(* Logix 5000 AddOnInstructionDefinition export GracoCore_DecodeDateTime; software revision 32.04 *)

TYPE GracoCore_TypeDateTime :
STRUCT
   year : DINT;   // year (yyyy)
   month : DINT;   // month (1=January, 2=February...12=December)
   dayOfMonth : DINT;   // day of the month (1-31)
   dayOfWeek : DINT;   // day of the week (1=Monday, 2=Tuesday...7=Sunday)
   hour : DINT;   // hour (0-23)
   min : DINT;   // min (0-59)
   sec : DINT;   // second (0-59)
END_STRUCT
END_TYPE

TYPE GracoPd2kDual_TypePd2kDualStatus :
STRUCT
   gunTriggerStatus1 : BOOL;   // gun 1 trigger status (1 = on)
   gunTriggerStatus2 : BOOL;   // gun 2 trigger status (1 = on)
   mixUnit1 : GracoPd2kDual_TypePd2kMixUnitStatus;   // mix unit 1
   mixUnit2 : GracoPd2kDual_TypePd2kMixUnitStatus;   // mix unit 2
   pump1 : GracoPd2kDual_TypePd2kPump;   // pump 1
   pump2 : GracoPd2kDual_TypePd2kPump;   // pump 2
   pump3 : GracoPd2kDual_TypePd2kPump;   // pump 3
   pump4 : GracoPd2kDual_TypePd2kPump;   // pump 4
   dcsReturn0 : DINT;   // DCS return 0
   dcsReturn1 : DINT;   // DCS return 1
   dcsReturn2 : DINT;   // DCS return 2
   dcsReturn3 : DINT;   // DCS return 3
   dcsReturn4 : DINT;   // DCS return 4
   dcsReturn5 : DINT;   // DCS return 5
   dcsReturn6 : DINT;   // DCS return 6
   dcsReturn7 : DINT;   // DCS return 7
   dcsReturn8 : DINT;   // DCS return 8
   dcsAck : DINT;   // DCS acknowledge
END_STRUCT
END_TYPE

TYPE GracoPd2kDual_TypePd2kMixUnitStatus :
STRUCT
   eventFlag : BOOL;   // event flag
   standby : BOOL;   // in standby
   interlockStatus : BOOL;   // interlock status
   systemMode : DINT;   // system mode
   systemModeFlags : GracoPd2kDual_TypePd2kSystemModeFlags;   // system mode flags
   actualMixFlow : DINT;   // actual mix flow (cc/min)
   actualMixRatio : DINT;   // actual mix ratio
   actualPotLifeRemaining : DINT;   // actual pot life remaining
   activeRecipeNum : DINT;   // active recipe number
   activeMaterialA : DINT;   // active material A
   activeMaterialB : DINT;   // active material B
   activeFlushSeqA : DINT;   // active flush sequence A
   activeFlushSeqB : DINT;   // active flush sequence B
   activeRatioSP : DINT;   // active ratio SP
   activePotLifeSP : DINT;   // active pot life SP
   activeJobNum : DINT;   // active job number
   jobSprayVolA : DINT;   // job sprayed volume A (cc)
   jobSprayVolB : DINT;   // job sprayed volume B (cc)
   jobSolventVol : DINT;   // job solvent volume used (cc)
END_STRUCT
END_TYPE

TYPE GracoPd2kDual_TypePd2kPump :
STRUCT
   status : DINT;   // pump status
   statusFlags : GracoPd2kDual_TypePd2kPumpStatusFlags;   // pump status flags
   actualMaterial : DINT;   // actual material number
   actualFlowRate : DINT;   // actual flow rate (cc/min)
   actualFluidPres : DINT;   // actual fluid pressure (psi)
END_STRUCT
END_TYPE

TYPE GracoPd2kDual_TypePd2kPumpStatusFlags :
STRUCT
   off : BOOL;   // off
   standby : BOOL;   // in standby
   busy : BOOL;   // busy
   flushing : BOOL;   // flushing
   priming : BOOL;   // priming
END_STRUCT
END_TYPE

TYPE GracoPd2kDual_TypePd2kSystemModeFlags :
STRUCT
   pumpOff : BOOL;   // pump off
   colorChange : BOOL;   // color change enabled
   colorChangePurgeA : BOOL;   // color change purging component A
   colorChangePurgeB : BOOL;   // color change purging component B
   colorChangeFilling : BOOL;   // color change filling
   mixFill : BOOL;   // mix fill
   mix : BOOL;   // mixing
   mixIdle : BOOL;   // mix idle
   purgeA : BOOL;   // purging component A
   purgeB : BOOL;   // purging component B
   standbyMixReady : BOOL;   // standby mix ready
   standbyFillReady : BOOL;   // standby fill ready
   standbyMixNotReady : BOOL;   // standby mix not ready
   standbyAlarm : BOOL;   // standby alarm
   lineFillingFlushing : BOOL;   // line is filling or flushing
   pumpPrimeFlush : BOOL;   // pump is priming or flushing
   maintCalibration : BOOL;   // maintenance/calibration
   mixSolventPush : BOOL;   // mix solvent push
END_STRUCT
END_TYPE

TYPE STRING4 :   // string type
STRUCT
   LEN : DINT;
   DATA : SINT[4];
END_STRUCT
END_TYPE

TYPE STRING9 :   // string type
STRUCT
   LEN : DINT;
   DATA : SINT[9];
END_STRUCT
END_TYPE

ADD_ON_INSTRUCTION GracoCore_DecodeDateTime   (* revision 1.0 *)
// Help:
// Convert from Graco-formatted date and time data into a UDT.
VAR_IN_OUT
   dateSource : DINT; {required}
   timeSource : DINT; {required}
   dateTimeDest : GracoCore_TypeDateTime; {required}
END_VAR
VAR
   buffer : DINT; {access None}
END_VAR

ROUTINE Logic   (* ladder *)
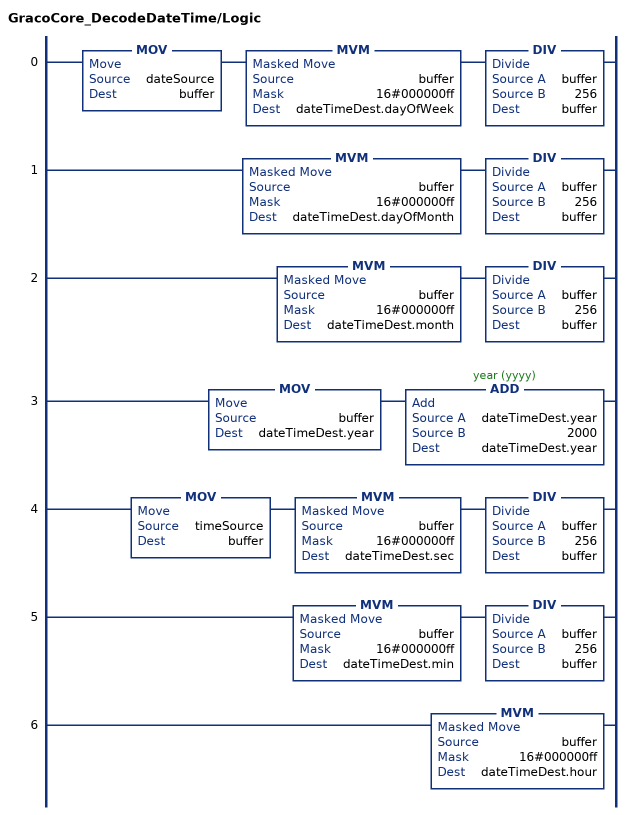
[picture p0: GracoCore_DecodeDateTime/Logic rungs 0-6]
   0: MOV(dateSource,buffer)MVM(buffer,16#000000ff,dateTimeDest.dayOfWeek)DIV(buffer,256,buffer);
   1: MVM(buffer,16#000000ff,dateTimeDest.dayOfMonth)DIV(buffer,256,buffer);
   2: MVM(buffer,16#000000ff,dateTimeDest.month)DIV(buffer,256,buffer);
   3: MOV(buffer,dateTimeDest.year)ADD(dateTimeDest.year,2000,dateTimeDest.year);
   4: MOV(timeSource,buffer)MVM(buffer,16#000000ff,dateTimeDest.sec)DIV(buffer,256,buffer);
   5: MVM(buffer,16#000000ff,dateTimeDest.min)DIV(buffer,256,buffer);
   6: MVM(buffer,16#000000ff,dateTimeDest.hour);
END_ROUTINE
END_ADD_ON_INSTRUCTION

ADD_ON_INSTRUCTION GracoCore_DecodeEventCode   (* revision 1.0 *)
// Help:
// Parses an event code String (max 4 characters) into a series of ASCII values stored in DINTs. These can then be written to a Graco CGM.
VAR_IN_OUT
   source : DINT; {required}
   dest : STRING4; {required}
END_VAR
VAR
   buffer : DINT; {access None}
END_VAR

ROUTINE Logic   (* ladder *)
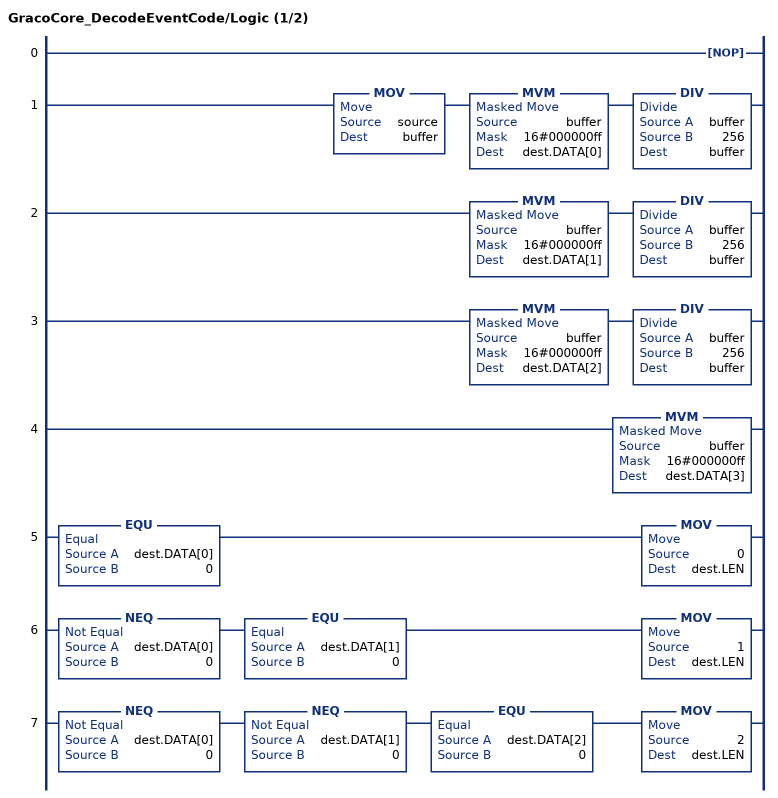
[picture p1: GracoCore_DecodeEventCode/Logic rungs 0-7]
   0: NOP();
   1: MOV(source,buffer)MVM(buffer,16#000000ff,dest.DATA[0])DIV(buffer,256,buffer);
   2: MVM(buffer,16#000000ff,dest.DATA[1])DIV(buffer,256,buffer);
   3: MVM(buffer,16#000000ff,dest.DATA[2])DIV(buffer,256,buffer);
   4: MVM(buffer,16#000000ff,dest.DATA[3]);
   5: EQU(dest.DATA[0],0)MOV(0,dest.LEN);
   6: NEQ(dest.DATA[0],0)EQU(dest.DATA[1],0)MOV(1,dest.LEN);
   7: NEQ(dest.DATA[0],0)NEQ(dest.DATA[1],0)EQU(dest.DATA[2],0)MOV(2,dest.LEN);
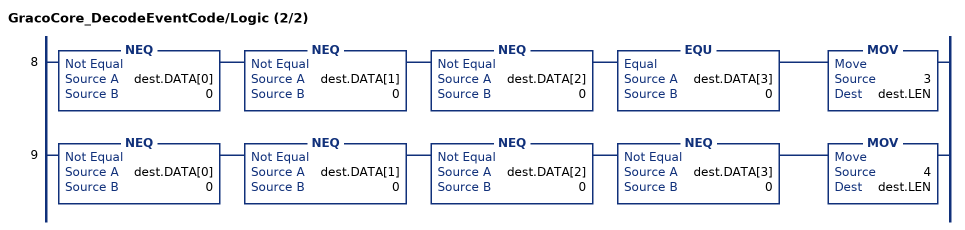
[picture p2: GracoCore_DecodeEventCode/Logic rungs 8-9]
   8: NEQ(dest.DATA[0],0)NEQ(dest.DATA[1],0)NEQ(dest.DATA[2],0)EQU(dest.DATA[3],0)MOV(3,dest.LEN);
   9: NEQ(dest.DATA[0],0)NEQ(dest.DATA[1],0)NEQ(dest.DATA[2],0)NEQ(dest.DATA[3],0)MOV(4,dest.LEN);
END_ROUTINE
END_ADD_ON_INSTRUCTION

ADD_ON_INSTRUCTION GracoPd2kDual_SendDCS   (* revision 1.0 *)
// Help:
// Sends a dynamic command structure (DCS) to the PD2K system.
// For more information about DCS commands, see the system operation manual.
// State Codes:
// * 0000 (IDLE) - Idle
// * 1000 (BUSY) - Busy
// * 2000 (DONE) - Done
// * 4000 (ABORT) - Command overwritten by another process
// * 8000 (ERROR) - Invalid command ID
// * 8001 (ERROR) - Timeout waiting for DCS registers
// * 8002 (ERROR) - Command unsuccessful
VAR_IN_OUT
   io_moduleStatus : DINT[62]; {required}   // Data from device to PLC
   io_moduleCmds : DINT[30]; {required}   // Data from PLC to device
END_VAR
VAR_INPUT
   i_execute : BOOL; {visible}   // Execute command
   i_cmdID : DINT; {visible}   // Command ID number
   i_arg0 : DINT; {visible}   // Argument 0
   i_arg1 : DINT; {visible}   // Argument 1
   i_arg2 : DINT; {visible}   // Argument 2
   i_arg3 : DINT; {visible}   // Argument 3
   i_arg4 : DINT; {visible}   // Argument 4
   i_arg5 : DINT; {visible}   // Argument 5
   i_arg6 : DINT; {visible}   // Argument 6
   i_arg7 : DINT; {visible}   // Argument 7
   i_arg8 : DINT; {visible}   // Argument 8
END_VAR
VAR_OUTPUT
   o_return0 : DINT; {access Read Only, visible}   // Return 0
   o_return1 : DINT; {access Read Only, visible}   // Return 1
   o_return2 : DINT; {access Read Only, visible}   // Return 2
   o_return3 : DINT; {access Read Only, visible}   // Return 3
   o_return4 : DINT; {access Read Only, visible}   // Return 4
   o_return5 : DINT; {access Read Only, visible}   // Return 5
   o_return6 : DINT; {access Read Only, visible}   // Return 6
   o_return7 : DINT; {access Read Only, visible}   // Return 7
   o_return8 : DINT; {access Read Only, visible}   // Return 8
   o_done : BOOL; {access Read Only, visible}   // Done flag
   o_busy : BOOL; {access Read Only, visible}   // Busy flag
   o_aborted : BOOL; {access Read Only, visible}   // Aborted flag
   o_error : BOOL; {access Read Only, visible}   // Error flag
   o_state : DINT; {access Read Only, visible}   // Command state
END_VAR
VAR
   _resetArgsTmr : TIMER := (PRE := 100); {access None}   // Reset arguments delay timer
   _inUseTmr : TIMER := (PRE := 5000); {access None}   // Register in use timer
   _sendArgsTmr : TIMER := (PRE := 100); {access None}   // Send arguments timer
   rateLimitTmr : TIMER := (PRE := 250); {access None}   // Rate limit timer
   cmdTimeoutTmr : TIMER := (PRE := 5000); {access None}   // Command timeout timer
   state_checkDcsReg : DINT; {access None}
   state_clearArgs : DINT; {access None}
   state_setArgs : DINT; {access None}
   state_setCmdID : DINT; {access None}
   state_awaitAck : DINT; {access None}
   state_rateLimit : DINT; {access None}
   state_done : DINT; {access None}
   state_aborted : DINT; {access None}
   state_invalidCmdID : DINT; {access None}
   state_dcsRegInUse : DINT; {access None}
   state_ackError : DINT; {access None}
   state_ackTimeout : DINT; {access None}
   initConfigValsDone : BOOL; {access None}
   _nextState : DINT; {access None}
   dcsRegAvailable : BOOL; {access None}
   _cmdID : DINT; {access None}
   execute_ons : BOOL; {access None}
END_VAR

ROUTINE Logic   (* ladder *)
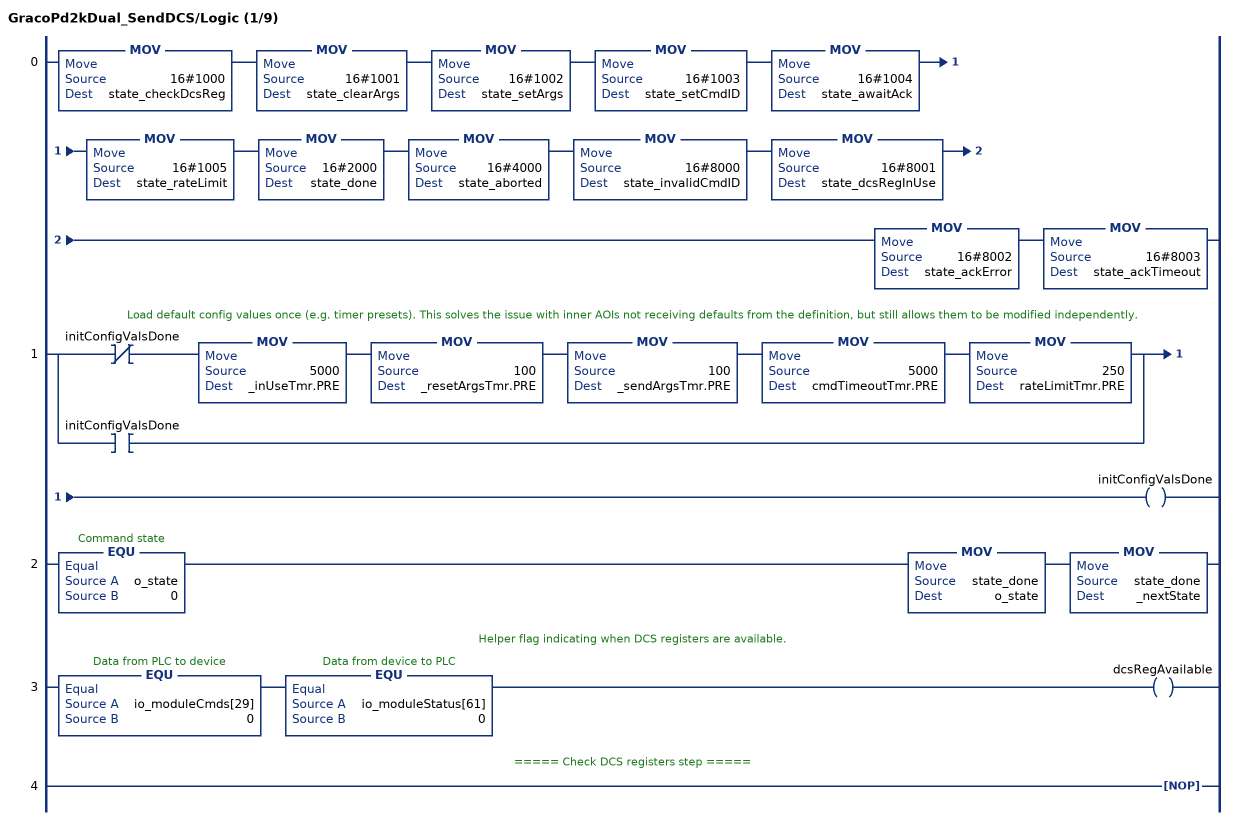
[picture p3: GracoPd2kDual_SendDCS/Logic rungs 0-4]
   0: MOV(16#1000,state_checkDcsReg)MOV(16#1001,state_clearArgs)MOV(16#1002,state_setArgs)MOV(16#1003,state_setCmdID)MOV(16#1004,state_awaitAck)MOV(16#1005,state_rateLimit)MOV(16#2000,state_done)MOV(16#4000,state_aborted)MOV(16#8000,state_invalidCmdID)MOV(16#8001,state_dcsRegInUse)MOV(16#8002,state_ackError)MOV(16#8003,state_ackTimeout);
   // Load default config values once (e.g. timer presets). This solves the issue with inner AOIs not receiving defaults from the definition, but still allows them to be modified independently.
   1: [XIO(initConfigValsDone) MOV(5000,_inUseTmr.PRE) MOV(100,_resetArgsTmr.PRE) MOV(100,_sendArgsTmr.PRE) MOV(5000,cmdTimeoutTmr.PRE) MOV(250,rateLimitTmr.PRE) ,XIC(initConfigValsDone) ]OTE(initConfigValsDone);
   2: EQU(o_state,0)MOV(state_done,o_state)MOV(state_done,_nextState);
   // Helper flag indicating when DCS registers are available.
   3: EQU(io_moduleCmds[29],0)EQU(io_moduleStatus[61],0)OTE(dcsRegAvailable);
   // ===== Check DCS registers step =====
   4: NOP();
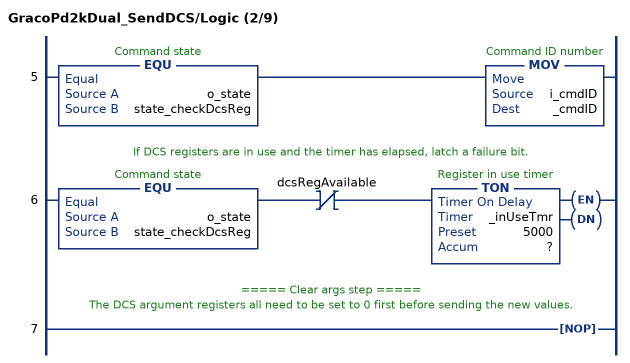
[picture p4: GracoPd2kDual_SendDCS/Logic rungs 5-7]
   5: EQU(o_state,state_checkDcsReg)MOV(i_cmdID,_cmdID);
   // If DCS registers are in use and the timer has elapsed, latch a failure bit.
   6: EQU(o_state,state_checkDcsReg)XIO(dcsRegAvailable)TON(_inUseTmr,?,?);
   // ===== Clear args step =====
   // The DCS argument registers all need to be set to 0 first before sending the new values.
   7: NOP();
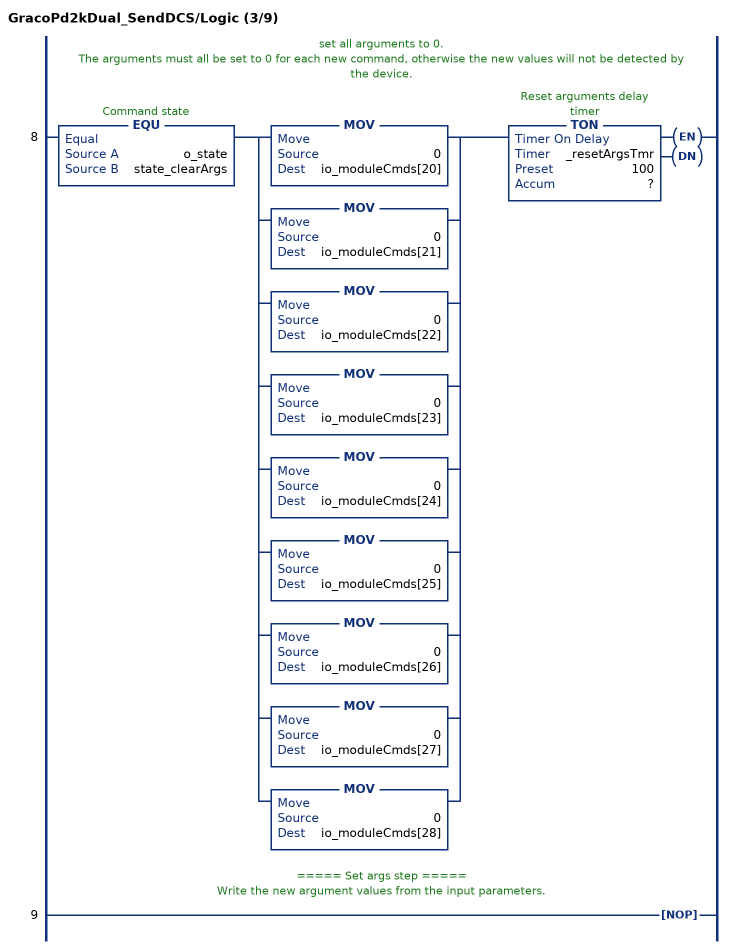
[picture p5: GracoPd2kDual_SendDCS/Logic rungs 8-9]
   // set all arguments to 0.
   // 		The arguments must all be set to 0 for each new command, otherwise the new values will not be detected by the device.
   8: EQU(o_state,state_clearArgs)[MOV(0,io_moduleCmds[20]) ,MOV(0,io_moduleCmds[21]) ,MOV(0,io_moduleCmds[22]) ,MOV(0,io_moduleCmds[23]) ,MOV(0,io_moduleCmds[24]) ,MOV(0,io_moduleCmds[25]) ,MOV(0,io_moduleCmds[26]) ,MOV(0,io_moduleCmds[27]) ,MOV(0,io_moduleCmds[28]) ]TON(_resetArgsTmr,?,?);
   // ===== Set args step =====
   // Write the new argument values from the input parameters.
   9: NOP();
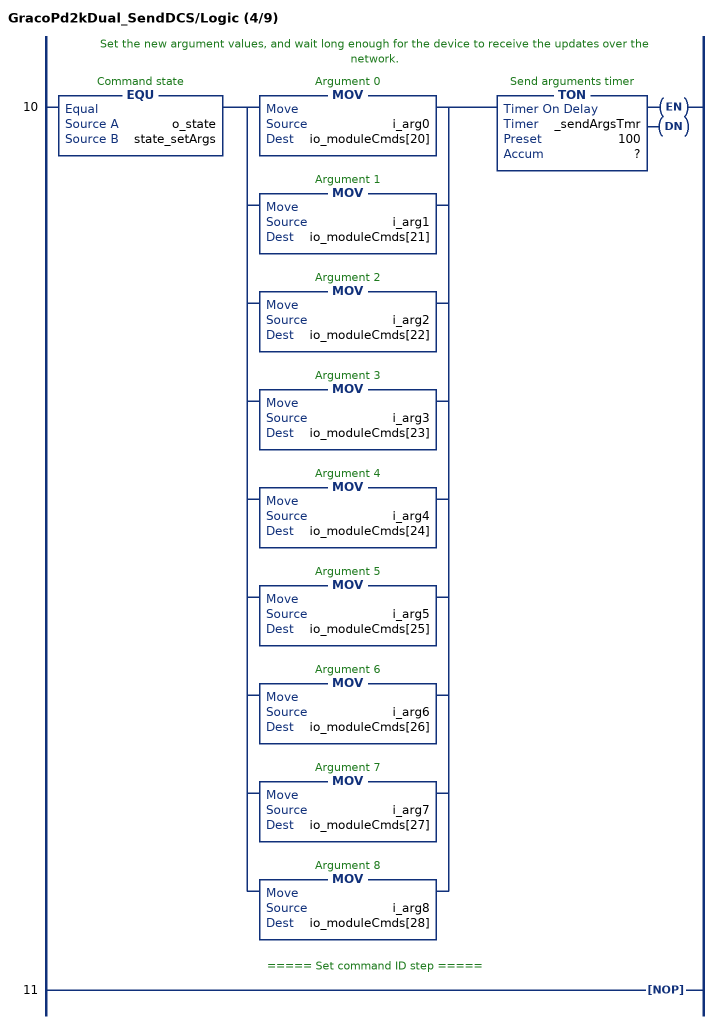
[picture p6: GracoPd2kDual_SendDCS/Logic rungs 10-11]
   // Set the new argument values, and wait long enough for the device to receive the updates over the network.
   10: EQU(o_state,state_setArgs)[MOV(i_arg0,io_moduleCmds[20]) ,MOV(i_arg1,io_moduleCmds[21]) ,MOV(i_arg2,io_moduleCmds[22]) ,MOV(i_arg3,io_moduleCmds[23]) ,MOV(i_arg4,io_moduleCmds[24]) ,MOV(i_arg5,io_moduleCmds[25]) ,MOV(i_arg6,io_moduleCmds[26]) ,MOV(i_arg7,io_moduleCmds[27]) ,MOV(i_arg8,io_moduleCmds[28]) ]TON(_sendArgsTmr,?,?);
   // ===== Set command ID step =====
   11: NOP();
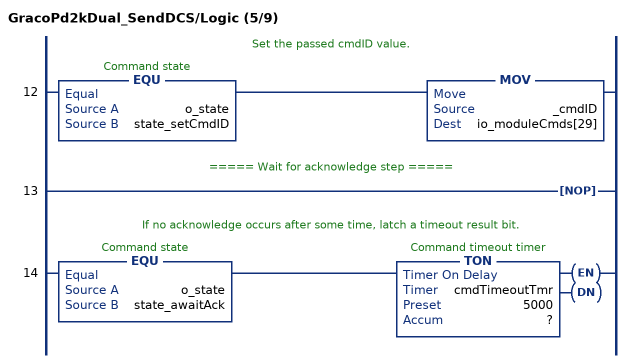
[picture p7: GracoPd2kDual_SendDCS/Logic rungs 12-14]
   // Set the passed cmdID value.
   12: EQU(o_state,state_setCmdID)MOV(_cmdID,io_moduleCmds[29]);
   // ===== Wait for acknowledge step =====
   13: NOP();
   // If no acknowledge occurs after some time, latch a timeout result bit.
   14: EQU(o_state,state_awaitAck)TON(cmdTimeoutTmr,?,?);
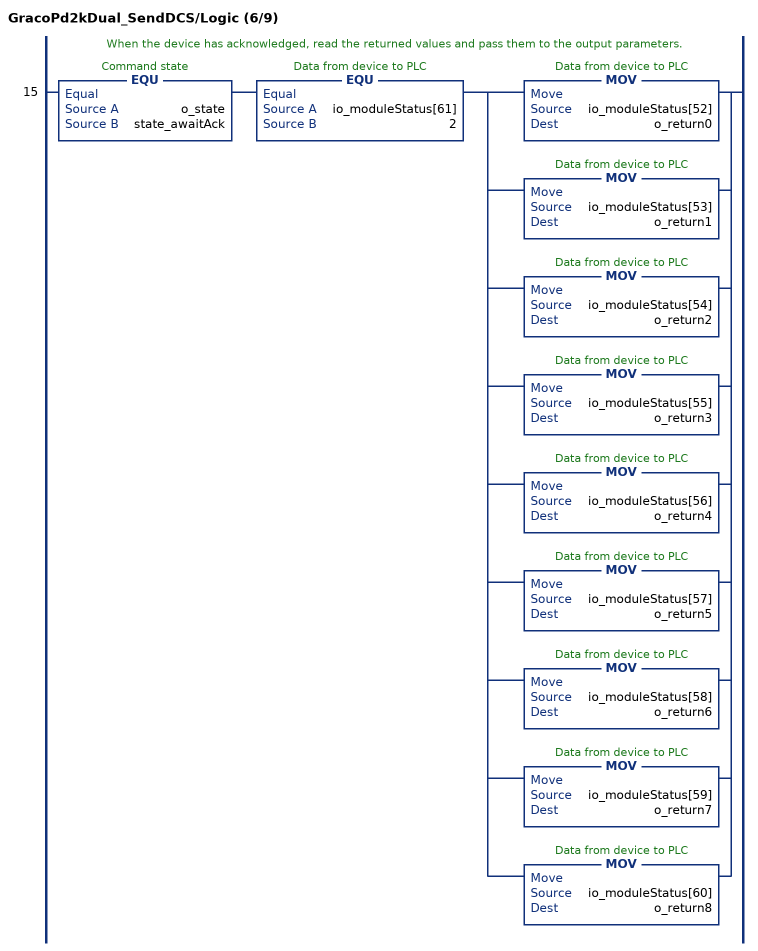
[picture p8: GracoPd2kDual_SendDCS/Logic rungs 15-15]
   // When the device has acknowledged, read the returned values and pass them to the output parameters.
   15: EQU(o_state,state_awaitAck)EQU(io_moduleStatus[61],2)[MOV(io_moduleStatus[52],o_return0) ,MOV(io_moduleStatus[53],o_return1) ,MOV(io_moduleStatus[54],o_return2) ,MOV(io_moduleStatus[55],o_return3) ,MOV(io_moduleStatus[56],o_return4) ,MOV(io_moduleStatus[57],o_return5) ,MOV(io_moduleStatus[58],o_return6) ,MOV(io_moduleStatus[59],o_return7) ,MOV(io_moduleStatus[60],o_return8) ];
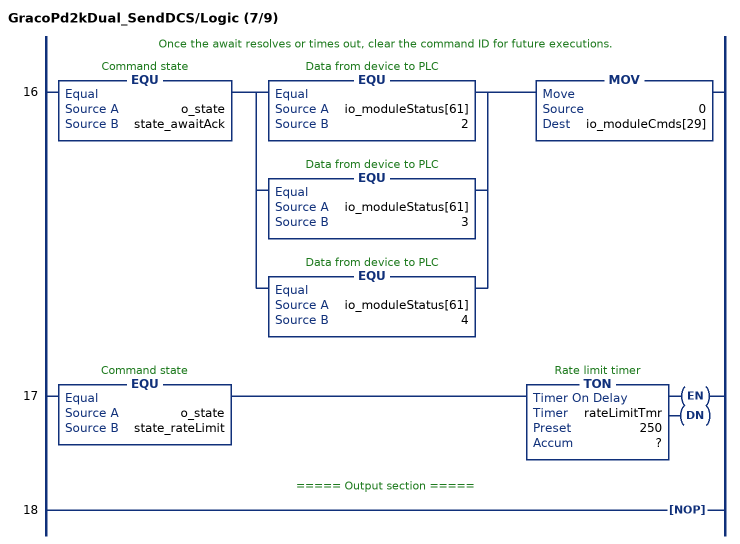
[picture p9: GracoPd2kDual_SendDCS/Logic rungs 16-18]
   // Once the await resolves or times out, clear the command ID for future executions.
   16: EQU(o_state,state_awaitAck)[EQU(io_moduleStatus[61],2) ,EQU(io_moduleStatus[61],3) ,EQU(io_moduleStatus[61],4) ]MOV(0,io_moduleCmds[29]);
   17: EQU(o_state,state_rateLimit)TON(rateLimitTmr,?,?);
   // ===== Output section =====
   18: NOP();
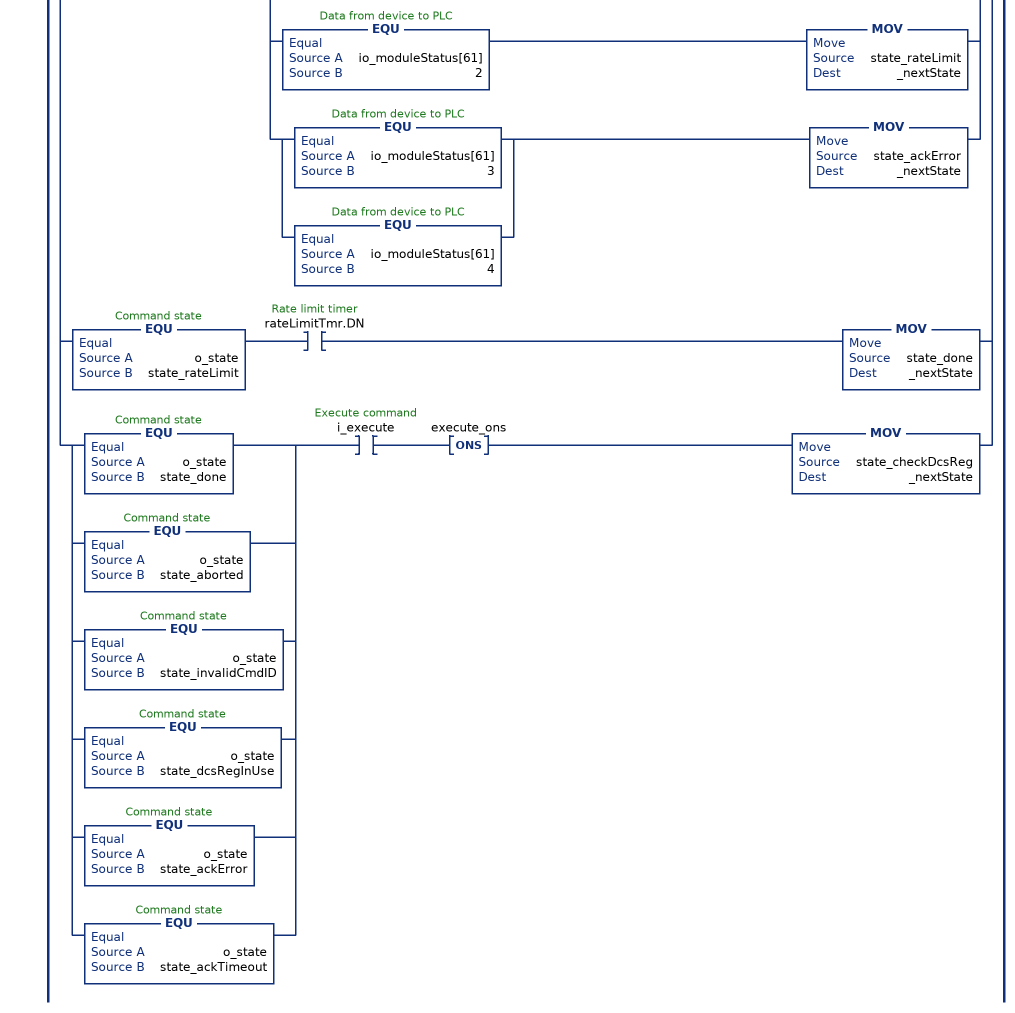
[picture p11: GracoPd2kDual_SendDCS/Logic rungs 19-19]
   19: [EQU(o_state,state_checkDcsReg) [EQU(_cmdID,0) MOV(state_invalidCmdID,_nextState) ,NEQ(_cmdID,0) [XIC(dcsRegAvailable) MOV(state_clearArgs,_nextState) ,XIC(_inUseTmr.DN) MOV(state_dcsRegInUse,_nextState) ] ] ,EQU(o_state,state_clearArgs) [XIO(dcsRegAvailable) MOV(state_checkDcsReg,_nextState) ,XIC(_resetArgsTmr.DN) MOV(state_setArgs,_nextState) ] ,EQU(o_state,state_setArgs) [XIO(dcsRegAvailable) MOV(state_checkDcsReg,_nextState) ,XIC(_sendArgsTmr.DN) MOV(state_setCmdID,_nextState) ] ,EQU(o_state,state_setCmdID) MOV(state_awaitAck,_nextState) ,EQU(o_state,state_awaitAck) [[EQU(io_moduleStatus[61],0) ,EQU(io_moduleStatus[61],1) ] [NEQ(io_moduleCmds[29],_cmdID) MOV(state_aborted,_nextState) ,XIC(cmdTimeoutTmr.DN) MOV(state_ackTimeout,_nextState) ] ,EQU(io_moduleStatus[61],2) MOV(state_rateLimit,_nextState) ,[EQU(io_moduleStatus[61],3) ,EQU(io_moduleStatus[61],4) ] MOV(state_ackError,_nextState) ] ,EQU(o_state,state_rateLimit) XIC(rateLimitTmr.DN) MOV(state_done,_nextState) ,[EQU(o_state,state_done) ,EQU(o_state,state_aborted) ,EQU(o_state,state_invalidCmdID) ,EQU(o_state,state_dcsRegInUse) ,EQU(o_state,state_ackError) ,EQU(o_state,state_ackTimeout) ] XIC(i_execute) ONS(execute_ons) MOV(state_checkDcsReg,_nextState) ];
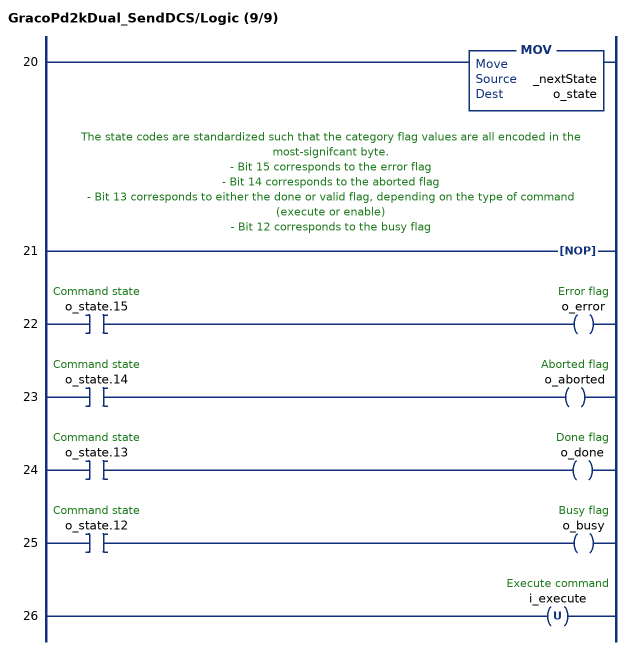
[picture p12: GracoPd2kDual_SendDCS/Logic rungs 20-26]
   20: MOV(_nextState,o_state);
   // The state codes are standardized such that the category flag values are all encoded in the most-signifcant byte.
   // - Bit 15 corresponds to the error flag
   // - Bit 14 corresponds to the aborted flag
   // - Bit 13 corresponds to either the done or valid flag, depending on the type of command (execute or enable)
   // - Bit 12 corresponds to the busy flag
   21: NOP();
   22: XIC(o_state.15)OTE(o_error);
   23: XIC(o_state.14)OTE(o_aborted);
   24: XIC(o_state.13)OTE(o_done);
   25: XIC(o_state.12)OTE(o_busy);
   26: OTU(i_execute);
END_ROUTINE
END_ADD_ON_INSTRUCTION

ADD_ON_INSTRUCTION GracoPd2kDual_ReadAlarmInfo   (* revision 1.0, vendor Graco Inc. *)
// Help:
// Returns data for an alarm record.
// If indexNum is out of range, an error will be raised.
// State Codes:
// * 0000 (IDLE) - Idle
// * 1000 (BUSY) - Busy
// * 2000 (DONE) - Done
// * 4000 (ABORT) - Command overwritten by another process
// * 8000 (ERROR) - Index number out of range
// * 8001 (ERROR) - Timeout waiting for DCS registers
// * 8002 (ERROR) - Command unsuccessful
// * 8003 (ERROR) - Unhandled internal error
VAR_INPUT
   i_execute : BOOL; {visible}   // Execute command
   i_indexNum : DINT; {visible}   // Index number
END_VAR
VAR_IN_OUT
   io_moduleStatus : DINT[62]; {required}   // Data from device to PLC
   io_moduleCmds : DINT[30]; {required}   // Data from PLC to device
   io_code : STRING4; {required}   // Alarm/event code
   io_dateTime : GracoCore_TypeDateTime; {required}   // Alarm/event datetime
END_VAR
VAR_OUTPUT
   o_busy : BOOL; {access Read Only, visible}   // Busy flag
   o_done : BOOL; {access Read Only, visible}   // Done flag
   o_aborted : BOOL; {access Read Only, visible}   // Aborted flag
   o_error : BOOL; {access Read Only, visible}   // Error flag
   o_state : DINT; {access Read Only, visible}   // Command state
END_VAR
VAR
   sendDCSInst : GracoPd2kDual_SendDCS; {access None}   // SendDCS instruction
   decodeDateTime : GracoCore_DecodeDateTime; {access None}   // DecodeDateTime instruction
   decodeEventCode : GracoCore_DecodeEventCode; {access None}   // DecodeEventCode instruction
END_VAR

ROUTINE Logic   (* ladder *)
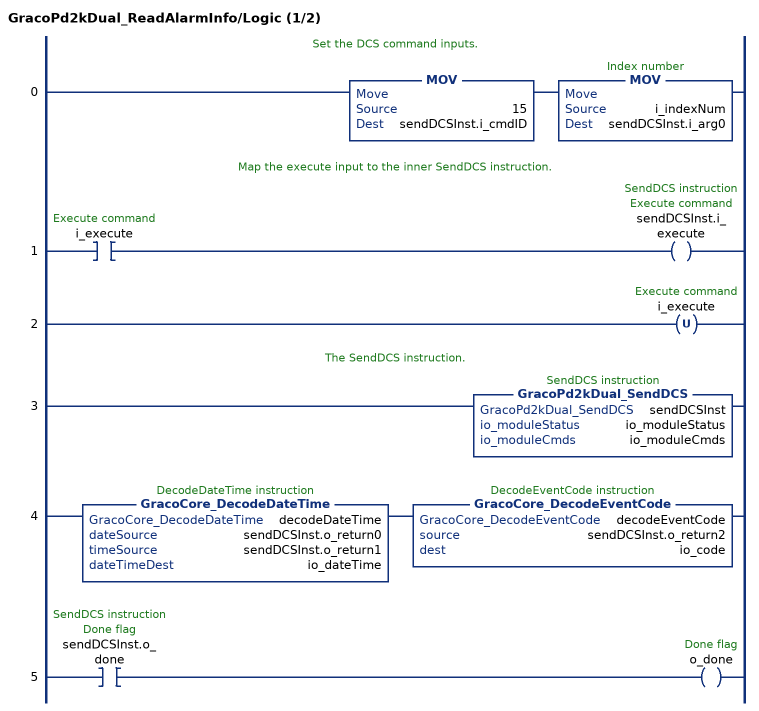
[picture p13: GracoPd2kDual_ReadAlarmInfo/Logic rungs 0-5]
   // Set the DCS command inputs.
   0: MOV(15,sendDCSInst.i_cmdID)MOV(i_indexNum,sendDCSInst.i_arg0);
   // Map the execute input to the inner SendDCS instruction.
   1: XIC(i_execute)OTE(sendDCSInst.i_execute);
   2: OTU(i_execute);
   // The SendDCS instruction.
   3: GracoPd2kDual_SendDCS(sendDCSInst,io_moduleStatus,io_moduleCmds);
   4: GracoCore_DecodeDateTime(decodeDateTime,sendDCSInst.o_return0,sendDCSInst.o_return1,io_dateTime)GracoCore_DecodeEventCode(decodeEventCode,sendDCSInst.o_return2,io_code);
   5: XIC(sendDCSInst.o_done)OTE(o_done);
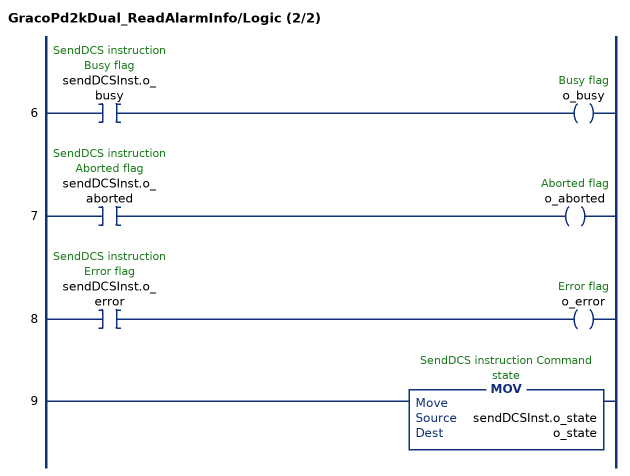
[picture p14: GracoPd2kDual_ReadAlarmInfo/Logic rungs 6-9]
   6: XIC(sendDCSInst.o_busy)OTE(o_busy);
   7: XIC(sendDCSInst.o_aborted)OTE(o_aborted);
   8: XIC(sendDCSInst.o_error)OTE(o_error);
   9: MOV(sendDCSInst.o_state,o_state);
END_ROUTINE
END_ADD_ON_INSTRUCTION

ADD_ON_INSTRUCTION GracoPd2kDual_ReadEventInfo   (* revision 1.0 *)
// Help:
// Returns data for an event record.
// If indexNum is out of range, an error will be raised.
// State Codes:
// * 0000 (IDLE) - Idle
// * 1000 (BUSY) - Busy
// * 2000 (DONE) - Done
// * 4000 (ABORT) - Command overwritten by another process
// * 8000 (ERROR) - Index number out of range
// * 8001 (ERROR) - Timeout waiting for DCS registers
// * 8002 (ERROR) - Command unsuccessful
// * 8003 (ERROR) - Unhandled internal error
VAR_INPUT
   i_execute : BOOL; {visible}   // Execute command
   i_indexNum : DINT; {visible}   // Index number
END_VAR
VAR_OUTPUT
   o_busy : BOOL; {access Read Only, visible}   // Busy flag
   o_done : BOOL; {access Read Only, visible}   // Done flag
   o_aborted : BOOL; {access Read Only, visible}   // Aborted flag
   o_error : BOOL; {access Read Only, visible}   // Error flag
   o_state : DINT; {access Read Only, visible}   // Command state
END_VAR
VAR_IN_OUT
   io_moduleStatus : DINT[62]; {required}   // Data from device to PLC
   io_moduleCmds : DINT[30]; {required}   // Data from PLC to device
   io_code : STRING4; {required}   // Alarm/event code
   io_dateTime : GracoCore_TypeDateTime; {required}   // Alarm/event datetime
END_VAR
VAR
   sendDCSInst : GracoPd2kDual_SendDCS; {access None}   // SendDCS instruction
   decodeDateTime : GracoCore_DecodeDateTime; {access None}   // DecodeDateTime instruction
   decodeEventCode : GracoCore_DecodeEventCode; {access None}   // DecodeEventCode instruction
END_VAR

ROUTINE Logic   (* ladder *)
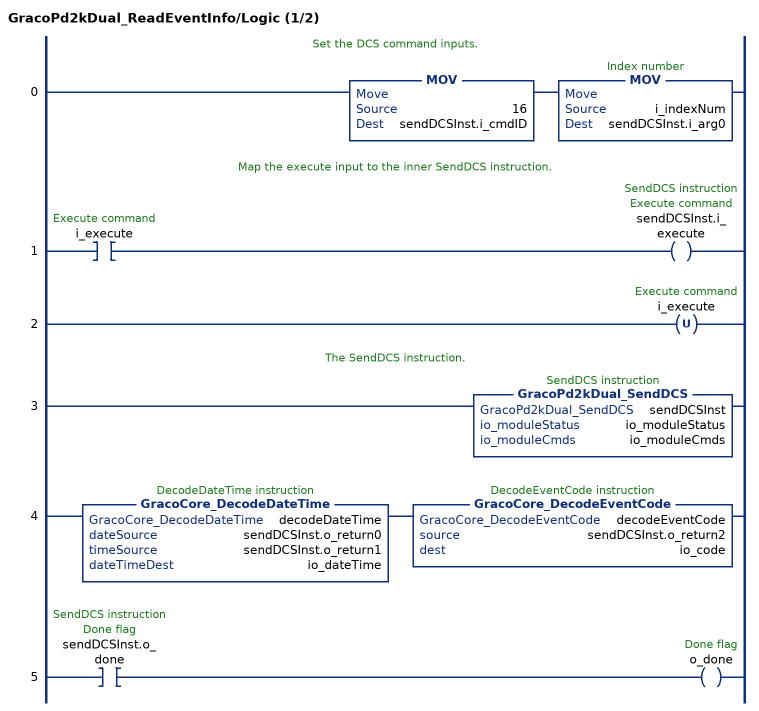
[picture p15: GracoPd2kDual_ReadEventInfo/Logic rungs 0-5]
   // Set the DCS command inputs.
   0: MOV(16,sendDCSInst.i_cmdID)MOV(i_indexNum,sendDCSInst.i_arg0);
   // Map the execute input to the inner SendDCS instruction.
   1: XIC(i_execute)OTE(sendDCSInst.i_execute);
   2: OTU(i_execute);
   // The SendDCS instruction.
   3: GracoPd2kDual_SendDCS(sendDCSInst,io_moduleStatus,io_moduleCmds);
   4: GracoCore_DecodeDateTime(decodeDateTime,sendDCSInst.o_return0,sendDCSInst.o_return1,io_dateTime)GracoCore_DecodeEventCode(decodeEventCode,sendDCSInst.o_return2,io_code);
   5: XIC(sendDCSInst.o_done)OTE(o_done);
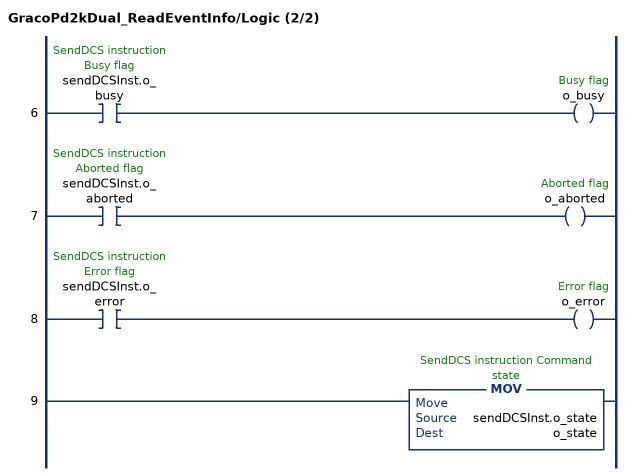
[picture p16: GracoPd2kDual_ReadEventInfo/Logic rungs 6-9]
   6: XIC(sendDCSInst.o_busy)OTE(o_busy);
   7: XIC(sendDCSInst.o_aborted)OTE(o_aborted);
   8: XIC(sendDCSInst.o_error)OTE(o_error);
   9: MOV(sendDCSInst.o_state,o_state);
END_ROUTINE
END_ADD_ON_INSTRUCTION

ADD_ON_INSTRUCTION GracoCore_DecodeUserID   (* revision 1.0 *)
// Help:
// Parses a user ID from a series of characters stored in DINTs into a Rockwell String (9 characters max).
VAR_IN_OUT
   source1 : DINT; {required}
   source2 : DINT; {required}
   source3 : DINT; {required}
   dest : STRING9; {required}
END_VAR
VAR
   buffer : DINT; {access None}
END_VAR

ROUTINE Logic   (* ladder *)
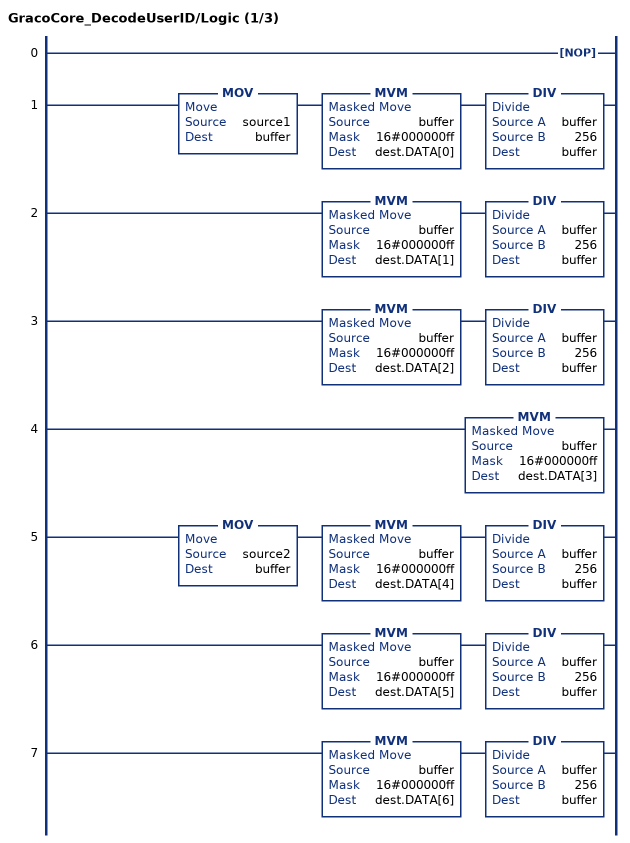
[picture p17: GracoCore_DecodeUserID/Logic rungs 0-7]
   0: NOP();
   1: MOV(source1,buffer)MVM(buffer,16#000000ff,dest.DATA[0])DIV(buffer,256,buffer);
   2: MVM(buffer,16#000000ff,dest.DATA[1])DIV(buffer,256,buffer);
   3: MVM(buffer,16#000000ff,dest.DATA[2])DIV(buffer,256,buffer);
   4: MVM(buffer,16#000000ff,dest.DATA[3]);
   5: MOV(source2,buffer)MVM(buffer,16#000000ff,dest.DATA[4])DIV(buffer,256,buffer);
   6: MVM(buffer,16#000000ff,dest.DATA[5])DIV(buffer,256,buffer);
   7: MVM(buffer,16#000000ff,dest.DATA[6])DIV(buffer,256,buffer);
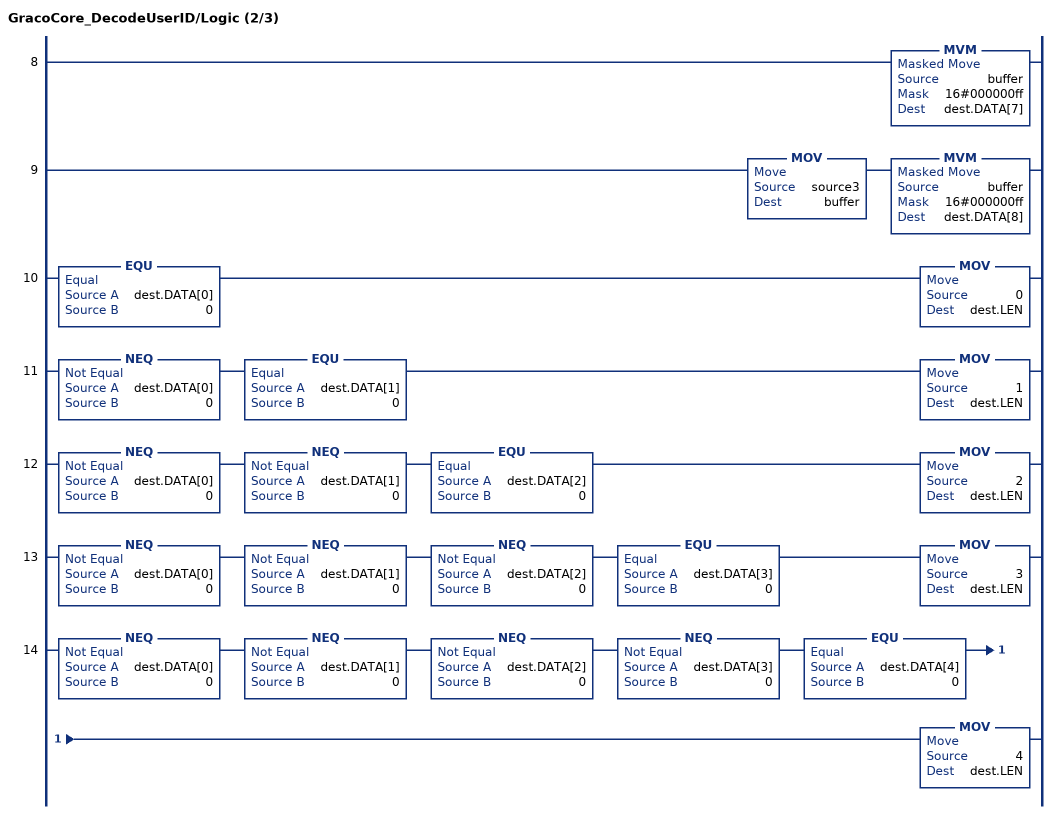
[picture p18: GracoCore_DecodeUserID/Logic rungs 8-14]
   8: MVM(buffer,16#000000ff,dest.DATA[7]);
   9: MOV(source3,buffer)MVM(buffer,16#000000ff,dest.DATA[8]);
   10: EQU(dest.DATA[0],0)MOV(0,dest.LEN);
   11: NEQ(dest.DATA[0],0)EQU(dest.DATA[1],0)MOV(1,dest.LEN);
   12: NEQ(dest.DATA[0],0)NEQ(dest.DATA[1],0)EQU(dest.DATA[2],0)MOV(2,dest.LEN);
   13: NEQ(dest.DATA[0],0)NEQ(dest.DATA[1],0)NEQ(dest.DATA[2],0)EQU(dest.DATA[3],0)MOV(3,dest.LEN);
   14: NEQ(dest.DATA[0],0)NEQ(dest.DATA[1],0)NEQ(dest.DATA[2],0)NEQ(dest.DATA[3],0)EQU(dest.DATA[4],0)MOV(4,dest.LEN);
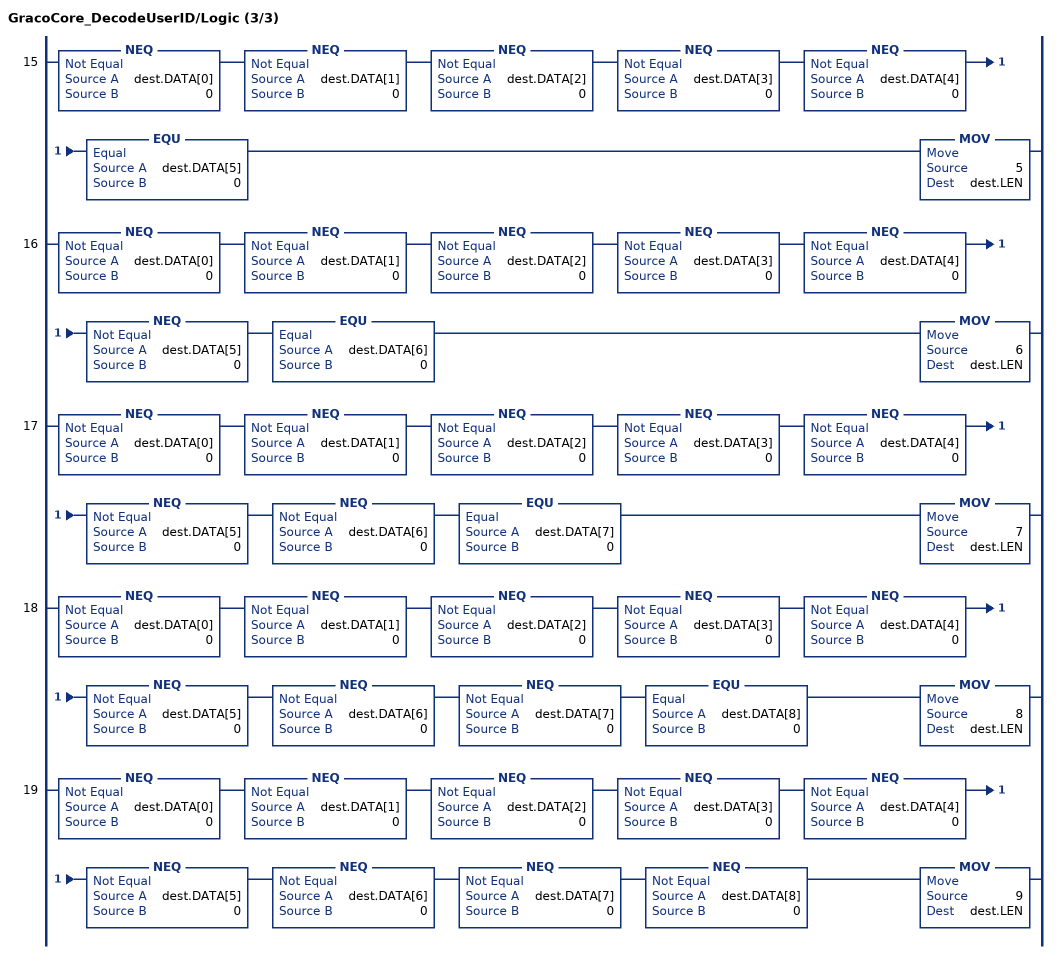
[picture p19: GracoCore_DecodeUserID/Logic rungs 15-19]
   15: NEQ(dest.DATA[0],0)NEQ(dest.DATA[1],0)NEQ(dest.DATA[2],0)NEQ(dest.DATA[3],0)NEQ(dest.DATA[4],0)EQU(dest.DATA[5],0)MOV(5,dest.LEN);
   16: NEQ(dest.DATA[0],0)NEQ(dest.DATA[1],0)NEQ(dest.DATA[2],0)NEQ(dest.DATA[3],0)NEQ(dest.DATA[4],0)NEQ(dest.DATA[5],0)EQU(dest.DATA[6],0)MOV(6,dest.LEN);
   17: NEQ(dest.DATA[0],0)NEQ(dest.DATA[1],0)NEQ(dest.DATA[2],0)NEQ(dest.DATA[3],0)NEQ(dest.DATA[4],0)NEQ(dest.DATA[5],0)NEQ(dest.DATA[6],0)EQU(dest.DATA[7],0)MOV(7,dest.LEN);
   18: NEQ(dest.DATA[0],0)NEQ(dest.DATA[1],0)NEQ(dest.DATA[2],0)NEQ(dest.DATA[3],0)NEQ(dest.DATA[4],0)NEQ(dest.DATA[5],0)NEQ(dest.DATA[6],0)NEQ(dest.DATA[7],0)EQU(dest.DATA[8],0)MOV(8,dest.LEN);
   19: NEQ(dest.DATA[0],0)NEQ(dest.DATA[1],0)NEQ(dest.DATA[2],0)NEQ(dest.DATA[3],0)NEQ(dest.DATA[4],0)NEQ(dest.DATA[5],0)NEQ(dest.DATA[6],0)NEQ(dest.DATA[7],0)NEQ(dest.DATA[8],0)MOV(9,dest.LEN);
END_ROUTINE
END_ADD_ON_INSTRUCTION
